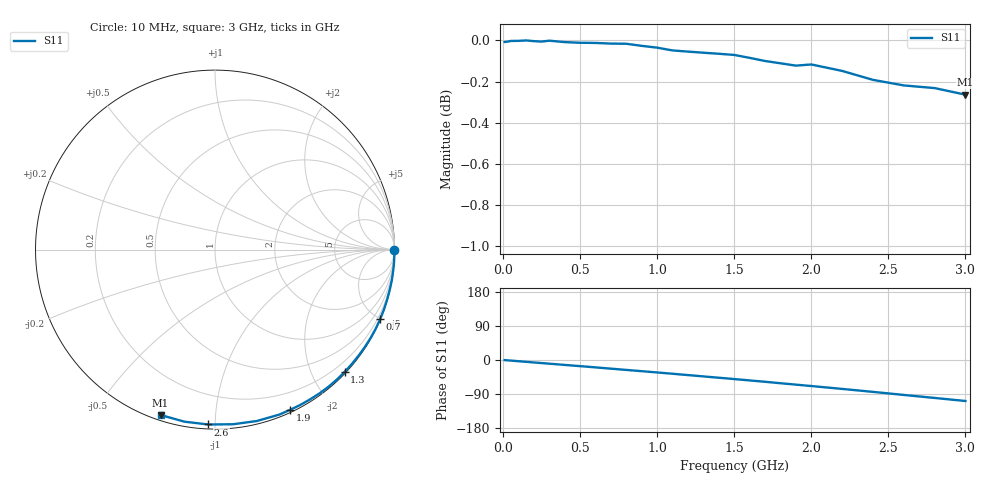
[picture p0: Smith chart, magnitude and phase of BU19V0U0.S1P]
! SIEMENS Small Signal Semiconductors
! BB833
! Si Tuning Diode in SOD323
! VR = 19 V
! S-Parameters:  April  1996
# GHz  S  MA  R  50
!  f  S11
! GHz  MAG  ANG
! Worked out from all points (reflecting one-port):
!   31 points, 10 MHz to 3 GHz, reference 50 ohm
!   lowest |S11| = -0.3 dB at 3 GHz (marker M1), VSWR 65.89, Z = 1.16 - j36.2 ohm
!   phase of S11 starts at -0 deg and turns -108 deg over the sweep
!   S11 on the Smith chart (normalised r, x): 10 MHz: open; 700 MHz: 0.02, -4.96; 1.3 GHz: 0.03, -2.52; 1.9 GHz: 0.02, -1.57; 2.6 GHz: 0.02, -0.96; 3 GHz: 0.02, -0.72
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0.01  0.9992 -0.2
0.02  0.9993 -0.6
0.05  0.9997 -1.6
0.15  1 -4.8
0.2  0.9996 -6.5
0.3  0.9999 -9.7
0.4  0.9991 -13.0
0.5  0.9987 -16.2
0.6  0.9986 -19.5
0.7  0.9982 -22.8
0.8  0.9981 -26.2
0.9  0.997 -29.5
1  0.996 -32.9
1.1  0.9944 -36.3
1.2  0.9938 -39.8
1.3  0.9931 -43.3
1.4  0.9926 -46.8
1.5  0.9919 -50.3
1.6  0.9903 -53.9
1.7  0.9886 -57.5
1.8  0.9873 -61.3
1.9  0.986 -65.0
2  0.9867 -68.7
2.2  0.9831 -76.3
2.4  0.9782 -84.1
2.6  0.9751 -92.2
2.8  0.9737 -100.1
3  0.9701 -108.2
